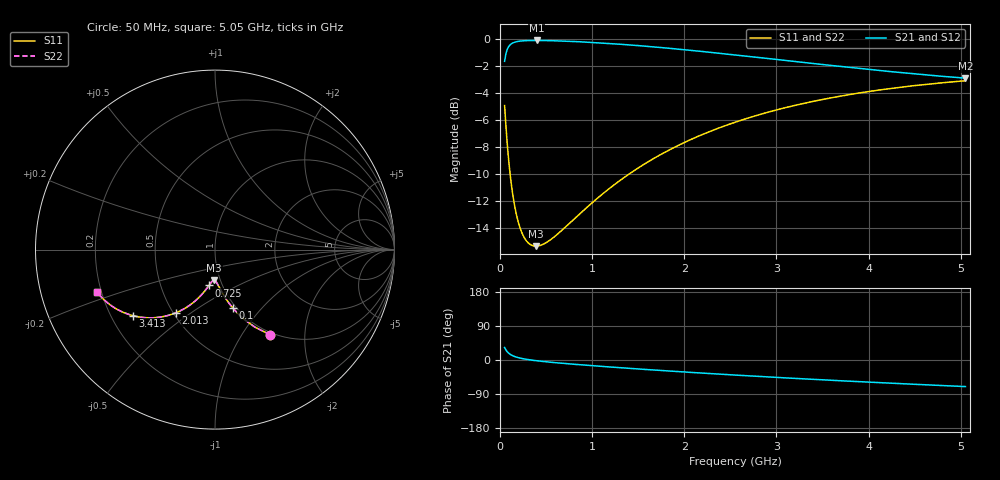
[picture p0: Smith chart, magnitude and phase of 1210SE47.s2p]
! AVX Thin Film Operation		Date: August 2001
! Description: Accu-P® Series, Thin Film, SMD, RF Capacitor
! Part Number: 12101J470FBT
! 50 MHz  -  5.05 GHz
! Serial Measurements
# mhz S db R 50
!	S11		S21		S12		S22
!	dB	Phase	dB	Phase	dB	Phase	dB	Phase
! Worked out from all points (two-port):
!   401 points, 50 MHz to 5.05 GHz, reference 50 ohm
!   highest |S21| = -0.13 dB at 400 MHz (marker M1); lowest = -2.9 dB at 5.05 GHz (marker M2)
!   |S21| within 3 dB of the highest: start of sweep to end of sweep
!   lowest |S11| = -15.4 dB at 387.5 MHz (marker M3), VSWR 1.41, Z = 46.7 - j16.4 ohm
!   |S11| at or under -10 dB: 109.3 MHz to 1.406 GHz (1.297 GHz wide, 171 % of centre)
!   |S22| runs from -15.4 to -3.1 dB; largest |S21 - S12| = 0
!   S11 on the Smith chart (normalised r, x): 50 MHz: 0.97, -1.35; 100 MHz: 0.96, -0.71; 725 MHz: 0.86, -0.36; 2.013 GHz: 0.51, -0.44; 3.413 GHz: 0.29, -0.33; 5.05 GHz: 0.18, -0.17
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50  -4.95 -57.0  -1.67 32.9  -1.67 32.9  -4.95 -57.0
75  -7.47 -67.2  -0.86 22.8  -0.86 22.8  -7.47 -67.2
87.5  -8.50 -70.5  -0.66 19.5  -0.66 19.5  -8.50 -70.5
100  -9.41 -73.1  -0.53 16.8  -0.53 16.8  -9.41 -73.2
125  -10.89 -77.1  -0.37 12.9  -0.37 12.9  -10.89 -77.1
150  -12.04 -79.9  -0.28 10.0  -0.28 10.0  -12.04 -79.9
175  -12.93 -82.1  -0.23 7.8  -0.23 7.8  -12.93 -82.1
212.5  -13.91 -84.6  -0.18 5.3  -0.18 5.3  -13.91 -84.6
287.5  -14.98 -88.2  -0.14 1.7  -0.14 1.7  -14.98 -88.2
387.5  -15.37 -91.6  -0.13 -1.7  -0.13 -1.7  -15.37 -91.6
400  -15.37 -92.0  -0.13 -2.0  -0.13 -2.0  -15.37 -92.0
525  -15.01 -95.2  -0.14 -5.3  -0.14 -5.3  -15.01 -95.2
725  -13.86 -99.6  -0.18 -9.7  -0.18 -9.7  -13.86 -99.6
887.5  -12.84 -102.8  -0.23 -12.9  -0.23 -12.9  -12.84 -102.8
1300  -10.51 -110.2  -0.41 -20.3  -0.41 -20.3  -10.51 -110.2
1725  -8.65 -117.3  -0.64 -27.3  -0.64 -27.3  -8.65 -117.3
2012.5  -7.65 -121.8  -0.82 -31.8  -0.82 -31.8  -7.65 -121.8
2550  -6.19 -129.7  -1.20 -39.7  -1.20 -39.7  -6.19 -129.7
3387.5  -4.66 -140.9  -1.83 -50.9  -1.83 -50.9  -4.66 -140.9
3412.5  -4.62 -141.2  -1.85 -51.3  -1.85 -51.3  -4.62 -141.2
4225  -3.70 -151.0  -2.43 -61.0  -2.43 -61.0  -3.70 -151.0
5050  -3.12 -160.1  -2.92 -70.2  -2.92 -70.2  -3.12 -160.1
